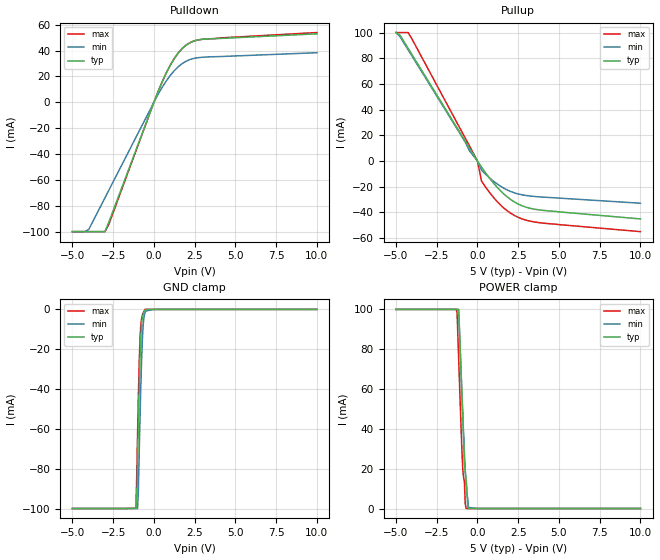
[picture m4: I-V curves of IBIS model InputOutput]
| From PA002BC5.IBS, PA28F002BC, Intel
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|********************Input Output Model 1**************************
[Model]   InputOutput
Model_type   I/O
|   Model for DQ[0:7] pins.
Vinl = 0.8V
Vinh = 2.0V
|Variable   Typ   Min   Max
C_comp   9.61p   NA   11.6p
[Voltage Range]   5.0V   4.5V   5.5V
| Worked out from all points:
|   slope of the pulldown table from 0 to 0.75 V, typ, clamps not added: 33.5 ohm
|   slope of the pullup table from 0 to 0.75 V, typ, clamps not added: 55.8 ohm
|   GND clamp passes 1 mA (typ) near -0.58 V on its own axis
|   POWER clamp passes 1 mA (typ) near -0.60 V on its own axis
[Pulldown]
| [Pullup] and [Pulldown] IV curves include only the current through
| the channels of output driver transistors when outputs are enabled
| with OE# = VIL.  Although the output driver transistors have np and
| pn diodes inherently created by CMOS IC fabrication between the
| drain and bulk of n-channel and p-channel CMOS transistors,
| the current through these junction diodes is not included in
| [Pullup] or [Pulldown].  Instead that drain/bulk diode current is
| included in the [POWER_clamp] or [GND_clamp] sections, which are
| not dependent on the state of OE# or output data value.
|Voltage   I(typ)   I(min)   I(max)
-5V       -100mA     -100mA     -100mA
-4.25V    -100mA     -100mA     -100mA
-4V       -100mA     -98.43mA   -100mA
-3V       -100mA     -73.83mA   -100mA
-2.75V    -92.23mA   -67.68mA   -93.86mA
0V        0A         0A         0A
500mV     15.52mA    11.36mA    15.52mA
1.25V     33.8mA     24.41mA    33.8mA
2V        44.4mA     31.9mA     44.4mA
2.5V      47.54mA    34.04mA    47.54mA
3V        48.72mA    34.82mA    48.72mA
10V       52.9mA     38.3mA     53.9mA
[GND_clamp]
| [POWER_clamp] and [GND_clamp] IV curves describe ESD protection
| circuits PLUS some np and pn diodes which exist between the
| drain and bulk of n-channel and p-channel CMOS transistors.
| These drain/bulk diodes are inherent in CMOS IC fabrication,
| and are visible on the node of the I/O pin at all times.
| Even the drain/bulk diodes of output driver [Pullup] and [Powerdown]
| transistors are included in [POWER_clamp] or [GND_clamp], because
| these diodes contribute to I/O pin current even when the
| chip outputs are tristated by OE# = VIH.
| For example, when V forced on the I/O pin is large, we are
| forward biasing the pn diode at the drain/bulk interface in the
| p-channel pullup transistor.  Similarly, when V forced on the
| I/O pin is sufficiently negative with respect to the substrate
| ground, we are forward biasing the np diode at the drain/bulk
| interface in the n-channel pulldown transistor.  The effects
| of these diodes are included in [POWER_clamp] or [GND_clamp].
|Voltage   I(typ)   I(min)   I(max)
-5V       -100mA     -100mA     -100mA
-1.1V     -100mA     -100mA     -99.84mA
-1.05V    -96mA      -100mA     -82.71mA
-1V       -75.49mA   -100mA     -61.98mA
-950mV    -56.26mA   -90.44mA   -42.74mA
-900mV    -38.64mA   -71.62mA   -26.37mA
-850mV    -24.17mA   -54.37mA   -14.4mA
-800mV    -13.03mA   -38.22mA   -7.425mA
-700mV    -3.595mA   -14.04mA   -2.781mA
-650mV    -2.149mA   -7.155mA   -1.713mA
-550mV    -639.7uA   -1.636mA   0A
10V       0A         0A         0A
[Pullup]
| (Voltages for [Pullup] and [POWER_clamp] are specified with
| negative respect to Vcc.  Reference the IBIS documentation
| for more information regarding Vtable = Vcc - Voutput.
| This method keeps -Vds constant for the values in all three
| columns across a line of the table.
| [Pullup] and [Pulldown] IV curves include only the current through
| the channels of output driver transistors when outputs are enabled
| with OE# = VIL.  Although the output driver transistors have np and
| pn diodes inherently created by CMOS IC fabrication between the
| drain and bulk of n-channel and p-channel CMOS transistors,
| the current through these junction diodes is not included in
| [Pullup] or [Pulldown].  Instead that drain/bulk diode current is
| included in the [POWER_clamp] or [GND_clamp] sections, which are
| not dependent on the state of OE# or output data value.
|Voltage  I(typ)   I(min)   I(max)
-5V       100mA      100mA      100mA
-4.75V    97.95mA    96.78mA    100mA
-4.25V    87.65mA    86.53mA    100mA
-750mV    15.55mA    14.78mA    17.9mA
-500mV    10.48mA    8.245mA    12.05mA
0V        0A         0A         0A
250mV     -4.65mA    -7.082mA   -15.57mA
1V        -17.38mA   -15.83mA   -28.53mA
1.75V     -27.07mA   -22mA      -37.94mA
2.5V      -33.44mA   -25.6mA    -43.79mA
3.5V      -37.44mA   -27.54mA   -47.4mA
10V       -45mA      -32.8mA    -54.9mA
[POWER_clamp]
| (Voltages for [Pullup] and [POWER_clamp] are specified with
| negative respect to Vcc.  Reference the IBIS documentation
| for more information regarding Vtable = Vcc - Voutput.
| This method keeps -Vds constant for the values in all three
| columns across a line of the table.
| [POWER_clamp] and [GND_clamp] IV curves describe ESD protection
| circuits PLUS some np and pn diodes which exist between the
| drain and bulk of n-channel and p-channel CMOS transistors.
| These drain/bulk diodes are inherent in CMOS IC fabrication,
| and are visible on the node of the I/O pin at all times.
| Even the drain/bulk diodes of output driver [Pullup] and [Powerdown]
| transistors are included in [POWER_clamp] or [GND_clamp], because
| these diodes contribute to I/O pin current even when the
| chip outputs are tristated by OE# = VIH.
| For example, when V forced on the I/O pin is large, we are
| forward biasing the pn diode at the drain/bulk interface in the
| p-channel pullup transistor.  Similarly, when V forced on the
| I/O pin is sufficiently negative with respect to the substrate
| ground, we are forward biasing the np diode at the drain/bulk
| interface in the n-channel pulldown transistor.  The effects
| of these diodes are included in [POWER_clamp] or [GND_clamp].
|Voltage I(typ)   I(min)   I(max)
-5V       100mA      100mA      100mA
-1.3V     100mA      100mA      100mA
-1.25V    100mA      100mA      98.33mA
-1.15V    100mA      98.06mA    74.61mA
-900mV    46.06mA    47.25mA    19.66mA
-800mV    22.5mA     27.99mA    13.36mA
-750mV    18.6mA     19.55mA    2.503mA
-700mV    14.56mA    12.38mA    68.4uA
-650mV    10.41mA    7.009mA    0A
-600mV    653.2uA    5.309mA    0A
-550mV    0A         538.8uA    0A
10V       0A         0A         0A
[Ramp]
| The DQ Ramp information is not provided at this time for the
| device but will be available in the future.  The table below
| is for the compatibility with some IBIS parsers.
| Variable   typ   min   max
 dV/dt_r   0V/0ns   0V/0ns   0V/0ns
 dV/dt_f   0V/0ns   0V/0ns   0V/0ns
